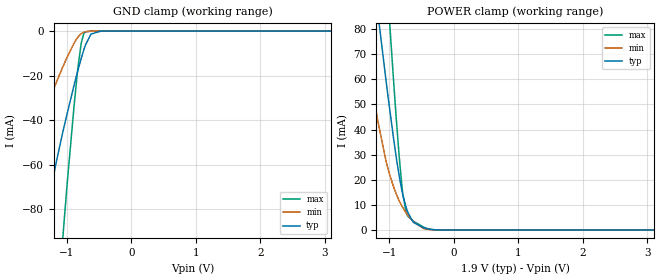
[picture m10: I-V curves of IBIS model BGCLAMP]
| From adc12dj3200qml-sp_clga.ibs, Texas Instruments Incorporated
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[Model]   BGCLAMP
Model_type   Terminator
|   typ   min   max
C_comp   1.17pF   1.09pF   1.25pF
[Voltage Range]   1.9   1.8   2
[Temperature Range]   25   125   -40
[Pullup Reference]   1.9   1.8   2
[Pulldown Reference]   0   0   0
[Power Clamp Reference]   1.9   1.8   2
[GND Clamp Reference]   0   0   0
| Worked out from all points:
|   GND clamp passes 1 mA (typ) near -0.59 V on its own axis
|   POWER clamp passes 1 mA (typ) near -0.48 V on its own axis
[GND Clamp]
|   Voltage   I(typ)   I(min)   I(max)
-1.9V     -241.6mA   -111.9mA   -561.3mA
-1.575V   -152.4mA   -60.14mA   -369.8mA
-1.359V   -96.95mA   -37.61mA   -244.7mA
-1.313V   -86.43mA   -34.13mA   -219mA
-1.205V   -65.33mA   -26.2mA    -159.9mA
-1.056V   -44.89mA   -15.84mA   -91.35mA
-839.8mV  -19.1mA    -3.239mA   -20.15mA
-777.1mV  -12.44mA   -1.195mA   -5.783mA
-737.2mV  -8.617mA   -514.4uA   -1.351mA
-623.2mV  -1.31mA    -28.37uA   -6.985uA
-469.3mV  -14.35uA   -454.5nA   -1.277uA
3.8V      0A         0A         0A
[POWER Clamp]
|   Voltage   I(typ)   I(min)   I(max)
-1.9V     249.8mA    157.2mA    461.7mA
-1.507V   159.9mA    93.42mA    292.9mA
-1.341V   122.7mA    67.61mA    223.2mA
-1.176V   86.38mA    43.35mA    155.1mA
-1.005V   50.5mA     23.07mA    86.94mA
-936.7mV  37.2mA     17.46mA    60.94mA
-885.4mV  28mA       14mA       42.49mA
-788.5mV  13.93mA    8.856mA    14.13mA
-714.4mV  7.199mA    6mA        5.628mA
-623.2mV  2.993mA    3.227mA    3.461mA
-469.3mV  889.7uA    617.6uA    1.156mA
3.8V      0A         0A         0A
